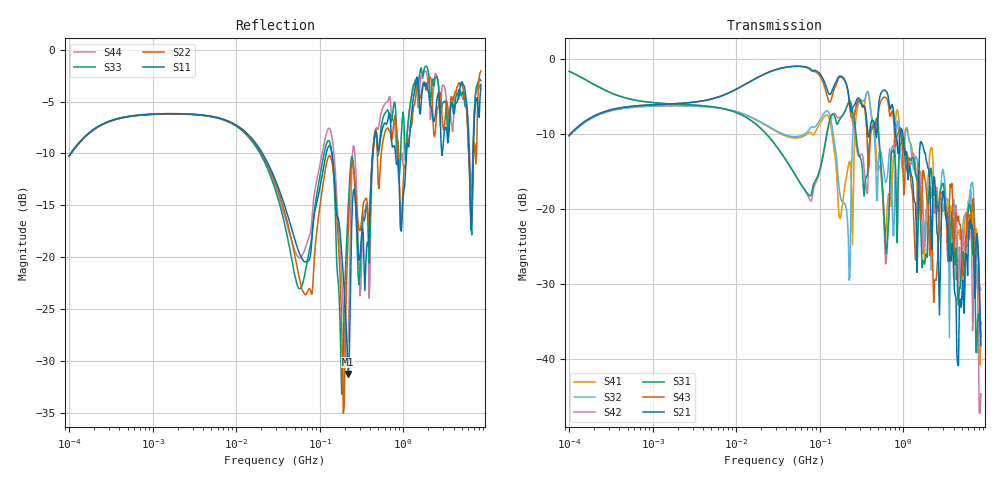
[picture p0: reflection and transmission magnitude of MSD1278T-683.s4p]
# MHz S MA R 50
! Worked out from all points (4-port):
!   498 points, 100 kHz to 8.5 GHz, reference 50 ohm
!   strongest paths, dB at 100 kHz, 1.698 MHz, 29.49 MHz, 500.7 MHz, 8.5 GHz:
!     S21: -10.2, -6.0, -1.4, -7.1, -38.3
!     S43: -10.2, -6.0, -1.4, -7.5, -37.1
!     S31: -1.6, -6.0, -11.5, -8.8, -35.1
!     S42: -1.6, -6.0, -11.4, -9.4, -44.7
!     S32: -10.3, -6.2, -9.5, -14.5, -30.8
!     S41: -10.3, -6.2, -9.6, -14.8, -36.7
!   lowest |S11| = -31.3 dB at 220 MHz (marker M1), VSWR 1.06, Z = 47.6 - j1.12 ohm
!   |S11| at or under -10 dB: 140 MHz to 432.6 MHz (292.6 MHz wide, 102 % of centre); 807.1 MHz to 1.092 GHz (285 MHz wide, 30 % of centre); 6.139 GHz to 6.867 GHz (727.8 MHz wide, 11.2 % of centre)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
0.1  0.3085 49.3  0.3099 50.2  0.8293 -16.8  0.3063 -130.5
     0.3099 50.2  0.3043 49.4  0.3063 -130.5  0.8301 -16.8
     0.8293 -16.8  0.3063 -130.5  0.3077 49.5  0.3107 50.1
     0.3063 -130.5  0.8301 -16.8  0.3107 50.1  0.3064 49.7
130.1252  0.3442 -39.0  0.5832 -35.1  0.3835 118.0  0.3998 -4.8
          0.5832 -35.1  0.3083 -30.3  0.4351 -8.8  0.3749 124.3
          0.3835 118.0  0.4351 -8.8  0.3628 -34.7  0.5165 -37.6
          0.3998 -4.8  0.3749 124.3  0.5165 -37.6  0.4179 -30.4
220.0307  0.02731 -154.5  0.5958 -66.6  0.5113 8.6  0.1943 22.1
          0.5958 -66.6  0.1373 41.8  0.06348 -11.1  0.5033 6.0
          0.5113 8.6  0.06348 -11.1  0.1775 29.1  0.5838 -72.4
          0.1943 22.1  0.5033 6.0  0.5838 -72.4  0.04328 35.8
372.0534  0.1177 64.1  0.3463 -81.9  0.1686 -18.8  0.6082 -37.4
          0.3463 -81.9  0.1811 48.4  0.6076 -41.8  0.1262 -22.7
          0.1686 -18.8  0.6076 -41.8  0.1694 23.8  0.2617 -100.4
          0.6082 -37.4  0.1262 -22.7  0.2617 -100.4  0.1718 9.2
2062.915  0.5653 173.8  0.1596 80.6  0.1571 -174.3  0.2258 171.6
          0.1596 80.6  0.7361 -176.8  0.08869 132.4  0.1197 155.0
          0.1571 -174.3  0.08869 132.4  0.6681 167.2  0.04865 -38.2
          0.2258 171.6  0.1197 155.0  0.04865 -38.2  0.5948 165.3
6173.935  0.2945 -168.1  0.08125 73.5  0.1076 112.1  0.1162 136.8
          0.08125 73.5  0.2794 -171.2  0.09726 134.3  0.08582 93.9
          0.1076 112.1  0.09726 134.3  0.2857 -165.5  0.06233 110.7
          0.1162 136.8  0.08582 93.9  0.06233 110.7  0.3569 -161.0
8500  0.6799 -49.9  0.01222 -118.8  0.01756 -75.0  0.01458 131.6
      0.01222 -118.8  0.7885 -42.3  0.02884 -130.7  0.005844 -65.1
      0.01756 -75.0  0.02884 -130.7  0.7087 -53.0  0.01399 13.3
      0.01458 131.6  0.005844 -65.1  0.01399 13.3  0.6435 -52.4
